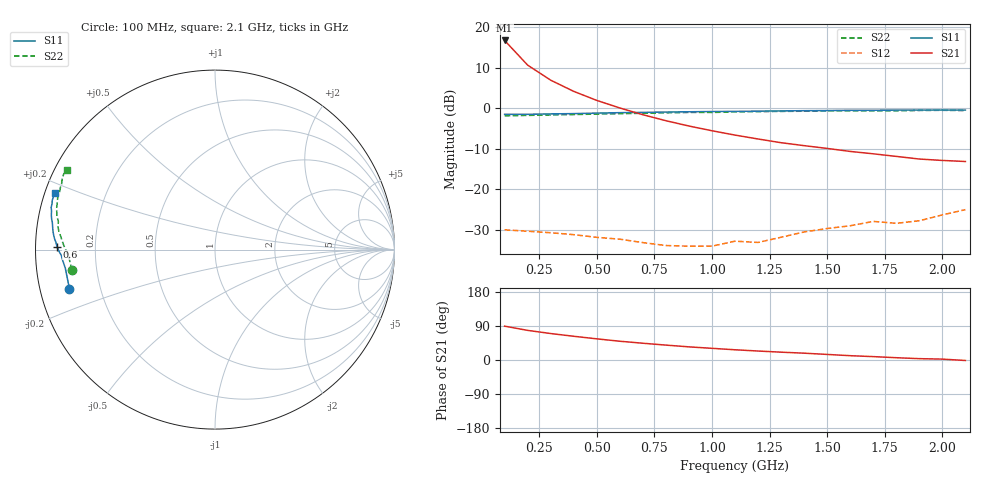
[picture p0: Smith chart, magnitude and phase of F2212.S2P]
! Date: Tue Aug 08 14:34:49 1995
# MHZ  S  MA  R  50.0000
!  POLYFET RF DEVICES
!  F2212
!  S PARAMETERS
!  VDS=12.5V, IDQ=800mA
!FREQ  S11MAG S11ANG S21MAG S21ANG S12MAG S12ANG S22MAG S22ANG
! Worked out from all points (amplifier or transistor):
!   21 points, 100 MHz to 2.1 GHz, reference 50 ohm
!   highest |S21| = 16.8 dB at 100 MHz (marker M1)
!   |S21| within 3 dB of that: start of sweep to 149.2 MHz
!   unconditionally stable (mu >= 1): 710 MHz to 1.341 GHz
!   at 400 MHz: K = 0.51, MSG = 17.7 dB, |S12| = -31.3 dB
!   at 1.1 GHz: K = 1.23, MAG = 10.2 dB, |S12| = -32.9 dB
!   at 2.1 GHz: K = 0.20, MSG = 6.0 dB, |S12| = -25.1 dB
!   S11 on the Smith chart (normalised r, x): 100 MHz: 0.09, -0.13; 600 MHz: 0.06, +0.01; 2.1 GHz: 0.03, +0.17
100  0.8399 -164.9  6.88 89.3  0.03138 3.9  0.8046 -171.9
200  0.8403 -172.9  3.408 78.2  0.03012 -1.7  0.8147 -176.7
300  0.8508 -176.0  2.221 69.9  0.02888 -5.2  0.8251 -178.8
400  0.857 -177.9  1.615 62.6  0.02732 -7.3  0.8349 179.6
500  0.8701 -179.5  1.249 55.8  0.02532 -6.0  0.8459 177.9
600  0.8807 178.9  1.006 49.5  0.02403 -4.6  0.856 176.2
700  0.8874 177.3  0.8305 44.2  0.02179 -2.3  0.8659 174.6
800  0.8962 176.1  0.7005 39.3  0.02005 4.4  0.8771 173.1
900  0.9036 174.6  0.6022 34.7  0.0197 8.1  0.8863 171.2
1000  0.9095 173.3  0.5263 30.8  0.01969 17.2  0.8859 170.0
1100  0.9139 171.9  0.4651 27.0  0.02269 24.2  0.8996 168.1
1200  0.9189 170.5  0.4163 23.7  0.02189 25.8  0.9074 166.4
1300  0.9255 169.5  0.3745 20.6  0.02537 32.7  0.9133 164.9
1400  0.9318 168.2  0.3443 18.0  0.02952 33.4  0.9179 163.2
1500  0.9356 166.8  0.3182 14.7  0.03255 32.4  0.9246 161.2
1600  0.9427 165.5  0.2922 11.4  0.03519 31.8  0.9237 159.7
1700  0.9431 164.3  0.273 8.9  0.03987 28.2  0.9284 158.0
1800  0.9472 163.2  0.2536 6.0  0.03773 26.3  0.9291 156.9
1900  0.9475 162.2  0.2352 3.6  0.0406 27.4  0.9374 155.3
2000  0.9491 161.3  0.226 2.3  0.04792 25.2  0.9422 153.5
2100  0.9477 160.5  0.2193 -1.3  0.05571 20.8  0.9343 151.7
